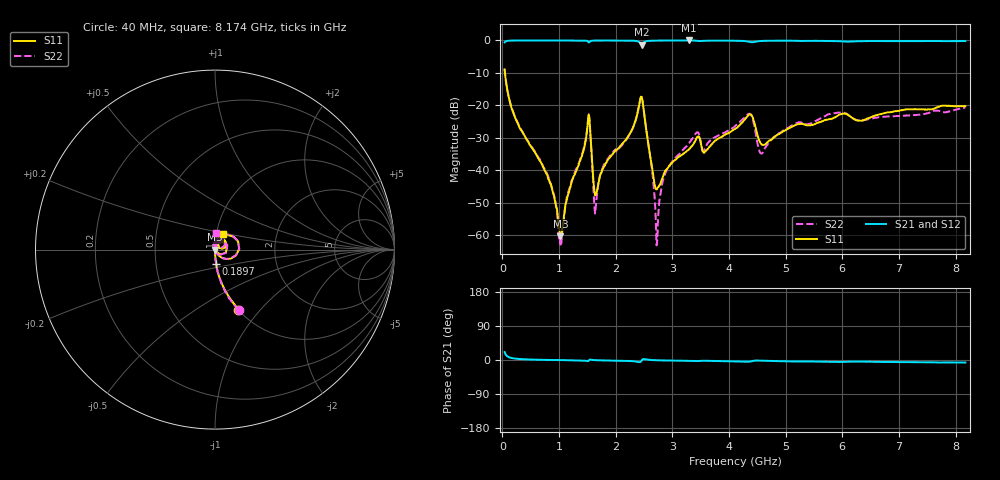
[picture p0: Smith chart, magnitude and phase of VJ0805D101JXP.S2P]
! VJ0805D101JXP
! DATE 10/29/2021  13:33
! CAPACITORS MOUNTED IN SERIES ON 25 MIL THICK MICROSTRIP SUBSTRATE
# GHz  S  MA  R  50.00
!  FREQ  S11M  S11A  S21M  S21A  S12M  S12A  S22M  S22A
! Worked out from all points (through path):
!   653 points, 40 MHz to 8.174 GHz, reference 50 ohm
!   highest |S21| = 0.00 dB at 3.296 GHz (marker M1); lowest = -1.3 dB at 2.46 GHz (marker M2)
!   group delay of S21, straight-line fit = 2.9 ps
!   lowest |S11| = -60.3 dB at 1.026 GHz (marker M3), VSWR 1.00, Z = 50.1 - j0.0325 ohm
!   |S11| at or under -10 dB: 46.24 MHz to end of sweep
!   |S22| runs from -63.3 to -8.8 dB; largest |S21 - S12| = 0.007
!   S11 on the Smith chart (normalised r, x): 40 MHz: 1.00, -0.77; 189.7 MHz: 1.00, -0.16; 8.174 GHz: 1.07, +0.19
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0.04  0.3582 -68.8  0.9354 21.0  0.9328 20.9  0.3636 -68.7
0.1897  0.078 -84.8  0.9967 4.4  0.996 4.4  0.07925 -85.7
0.800975  0.007985 -86.5  0.9982 0.3  0.9997 0.2  0.008464 -90.4
1.025525  0.0009649 -19.6  0.9988 -0.3  0.9993 -0.3  0.0006895 -28.0
1.175225  0.004601 74.3  0.9986 -0.6  0.9991 -0.6  0.004951 82.0
1.399775  0.01622 78.9  0.9963 -1.3  0.9978 -1.4  0.01721 81.5
1.524525  0.0718 20.4  0.9318 -2.0  0.9333 -2.1  0.0736 19.9
1.649275  0.004192 19.4  0.9964 -0.6  0.9979 -0.6  0.002744 46.4
1.7865  0.01111 71.8  0.9972 -1.1  0.9983 -1.2  0.01194 85.9
2.248075  0.03644 81.0  0.9944 -2.7  0.9958 -2.7  0.03561 83.1
2.46015  0.1351 1.1  0.8649 -1.1  0.8666 -1.2  0.1351 2.9
2.6348  0.01235 -52.0  0.991 -0.1  0.9932 -0.2  0.01154 -68.7
2.70965  0.005203 -7.0  0.9941 -0.6  0.9969 -0.7  0.001552 -48.8
2.75955  0.005593 27.5  0.9954 -0.9  0.9975 -1.0  0.002531 87.5
2.8843  0.01011 62.6  0.9971 -1.3  0.9978 -1.3  0.009493 101.7
3.295975  0.02119 77.7  0.9999 -2.3  1.001 -2.4  0.02624 103.9
4.119325  0.04401 72.2  0.9911 -3.6  0.9935 -3.7  0.0491 88.7
4.3813  0.0731 35.7  0.9435 -3.9  0.9451 -4.1  0.0737 44.7
4.568425  0.02576 26.5  0.9822 -1.8  0.9831 -1.9  0.01823 53.9
5.466625  0.05004 53.8  0.9852 -4.0  0.9878 -4.2  0.05367 91.4
6.8264  0.07838 59.6  0.9775 -5.3  0.9797 -5.5  0.06776 78.7
8.1737  0.09747 63.4  0.9788 -6.8  0.9817 -7.1  0.09339 85.1
